(* Logix 5000 AddOnInstructionDefinition export Banner_TL50_Param_v4; software revision 32.00 *)

TYPE Banner_IOL_Port_v4 :   // UDT that has all of the data items necessary to communicate with a specific Port on a IO-Link Master
STRUCT
   Port_Controlled : INT;   // Each bit represents a port on an IO-Link Master. Set to 1 to tell AOI to control that port.
   Port_Activate : INT;   // Each bit represents a port on an IO-Link Master. When ON that port will process any commands in queue.
   Port_Read : INT;   // Each bit represents a port on an IO-Link Master. Used to determine when device AOI has requested a Read command.
   Port_Write : INT;   // Each bit represents a port on an IO-Link Master. Used to determine when device AOI has requested a Write command.
   Port_RW_Complete : INT;   // Each bit represents a port on an IO-Link Master. Tells device AOI that Read or Write request has been completed.
   Port_Device_Read : INT;
   Data_Transfer : SINT[190];   // Array to transfer data from IO-Master to device AOIs.
END_STRUCT
END_TYPE

TYPE Banner_TL50_RD_v2 :   // All of the read parameters for a TL50.
STRUCT
   Master_Cycle_Time : INT;
   Min_Cycle_Time : INT;
   M_Sequence_Capability : INT;
   IO_Link_Version_ID : INT;
   Process_Data_Input_Length : INT;
   Process_Data_Output_Length : INT;
   Combined_Vendor_ID : DINT;   // IO-Link Vendor ID
   Vendor_ID1 : INT;
   Vendor_ID2 : INT;
   Combined_Device_ID : DINT;   // IO-Link Device ID
   Device_ID1 : INT;
   Device_ID2 : INT;
   Device_ID3 : INT;
   Serial_Number : STRING;
   Segment_1_State : SINT;   // State of the TL50 Segment. 0 = Off, 1 = On, 2 = Flashing
   Segment_2_State : SINT;   // State of the TL50 Segment. 0 = Off, 1 = On, 2 = Flashing
   Segment_3_State : SINT;   // State of the TL50 Segment. 0 = Off, 1 = On, 2 = Flashing
   Segment_4_State : SINT;   // State of the TL50 Segment. 0 = Off, 1 = On, 2 = Flashing
   Segment_5_State : SINT;   // State of the TL50 Segment. 0 = Off, 1 = On, 2 = Flashing
   Segment_6_State : SINT;   // State of the TL50 Segment. 0 = Off, 1 = On, 2 = Flashing
   Segment_7_State : SINT;   // State of the TL50 Segment. 0 = Off, 1 = On, 2 = Flashing
   Number_of_Segments : INT;   // Number of Segment detected for the TL50.
END_STRUCT
END_TYPE

TYPE Banner_TL50_v2 :   // All of the parameters for a TL50.
STRUCT
   Initial_Global_Read : BOOL;   // Determines if all of the IO-Link data has been read into the PLC yet
   Command : INT;   // Value placed in here will activate a read or write to a specifc IO-Link Index
   Read_Data : Banner_TL50_RD_v2;   // Read Only Data
   Write_Data : Banner_TL50_WD_v2;   // Write Data
   Archive : Banner_TL50_WD_v2;   // Archive Data
   Reset : BOOL;   // Resets AOI. This will force a complete parameter read of the sensor.
END_STRUCT
END_TYPE

TYPE Banner_TL50_WD_v2 :   // UDT that stores the Write Data for a TL50.
STRUCT
   System_Command : INT;   // See IODD file for list of commands that can be activated via the System Command interface
   Parameter_Access_Lock : SINT;   // Write access to all parameters is prohibited while value is 1. Only this parameter can be adjusted when value is 1.
   Data_Storage_Lock : SINT;   // Automatic data storage is disabled when this value is equal to 1. Read access is not affected.
   Local_Parameterization_Lock : SINT;   // Parameterization via local control elements on device is disabled.
   Local_User_Interface_Lock : SINT;   // Operation of local user interface is disabled.
   Flashing_Frequency_1 : DINT;   // Value in .1 Hz increments.
   Flashing_Frequency_2 : DINT;   // Value in .1 Hz increments.
   Flashing_Frequency_3 : DINT;   // Value in .1 Hz increments.
   Flashing_Frequency_4 : DINT;   // Value in .1 Hz increments.
   Flashing_Frequency_5 : DINT;   // Value in .1 Hz increments.
   Flashing_Frequency_6 : DINT;   // Value in .1 Hz increments.
   Flashing_Frequency_7 : DINT;   // Value in .1 Hz increments.
END_STRUCT
END_TYPE

ADD_ON_INSTRUCTION Banner_TL50_Param_v4   (* revision 4.0, vendor Banner Engineering *)
// AOI to read and write parameter data to an IO-Link TL50.
VAR_IN_OUT
   TL50 : Banner_TL50_v2; {required}
   Port_Data : Banner_IOL_Port_v4; {required}
END_VAR
VAR_INPUT
   Port : DINT; {required}
END_VAR
VAR
   Local_Control : DINT; {access None}
   Global_Read_Command_Value : INT; {access None}
   Global_Write_Command_Value : INT; {access None}
   Error_Generated : BOOL; {access None}
   Command_Being_Processed : BOOL; {access None}
   Index_Write_Inprocess : INT; {access None}
   Index_Write_Control : INT; {access None}
   Update_Archive : BOOL; {access None}
   Inprocess_Index : DINT; {access None}
END_VAR

ROUTINE Logic   (* ladder *)
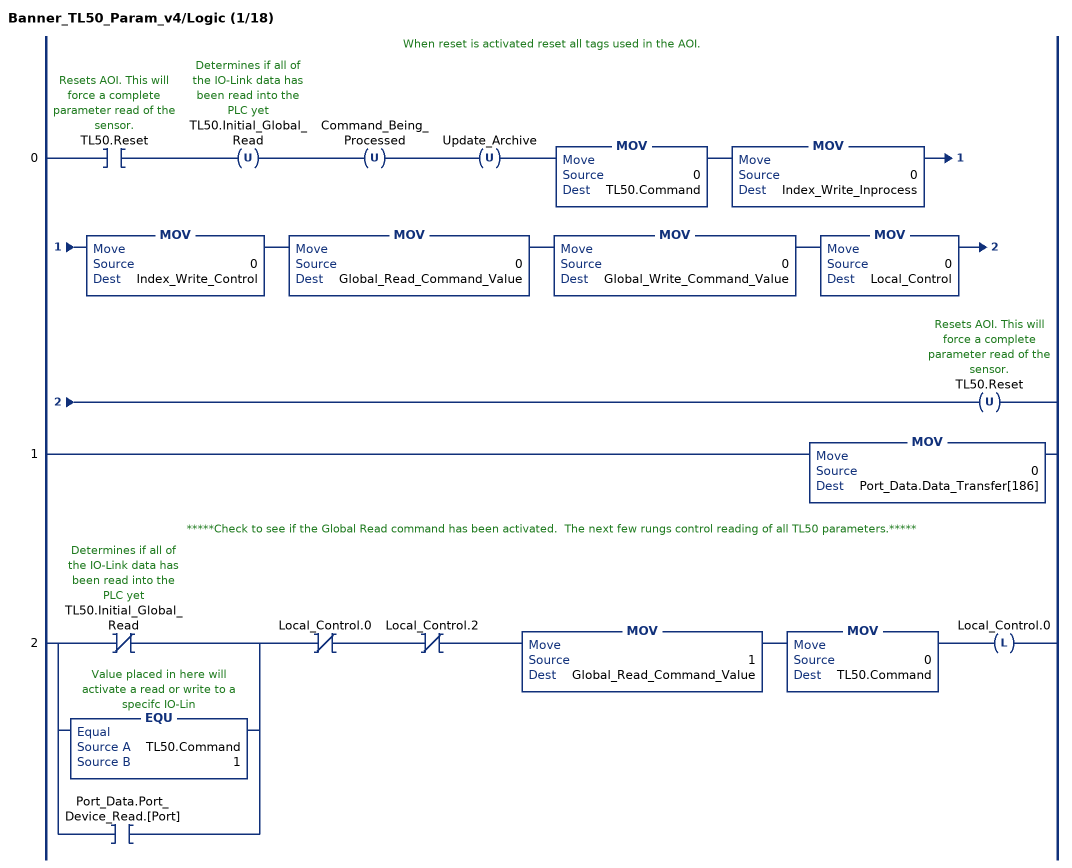
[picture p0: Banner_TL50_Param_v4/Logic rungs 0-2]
   // When reset is activated reset all tags used in the AOI.
   0: XIC(TL50.Reset)OTU(TL50.Initial_Global_Read)OTU(Command_Being_Processed)OTU(Update_Archive)MOV(0,TL50.Command)MOV(0,Index_Write_Inprocess)MOV(0,Index_Write_Control)MOV(0,Global_Read_Command_Value)MOV(0,Global_Write_Command_Value)MOV(0,Local_Control)OTU(TL50.Reset);
   1: MOV(0,Port_Data.Data_Transfer[186]);
   // *****Check to see if the Global Read command has been activated.  The next few rungs control reading of all TL50 parameters.*****
   2: [XIO(TL50.Initial_Global_Read) ,EQU(TL50.Command,1) ,XIC(Port_Data.Port_Device_Read.[Port]) ]XIO(Local_Control.0)XIO(Local_Control.2)MOV(1,Global_Read_Command_Value)MOV(0,TL50.Command)OTL(Local_Control.0);
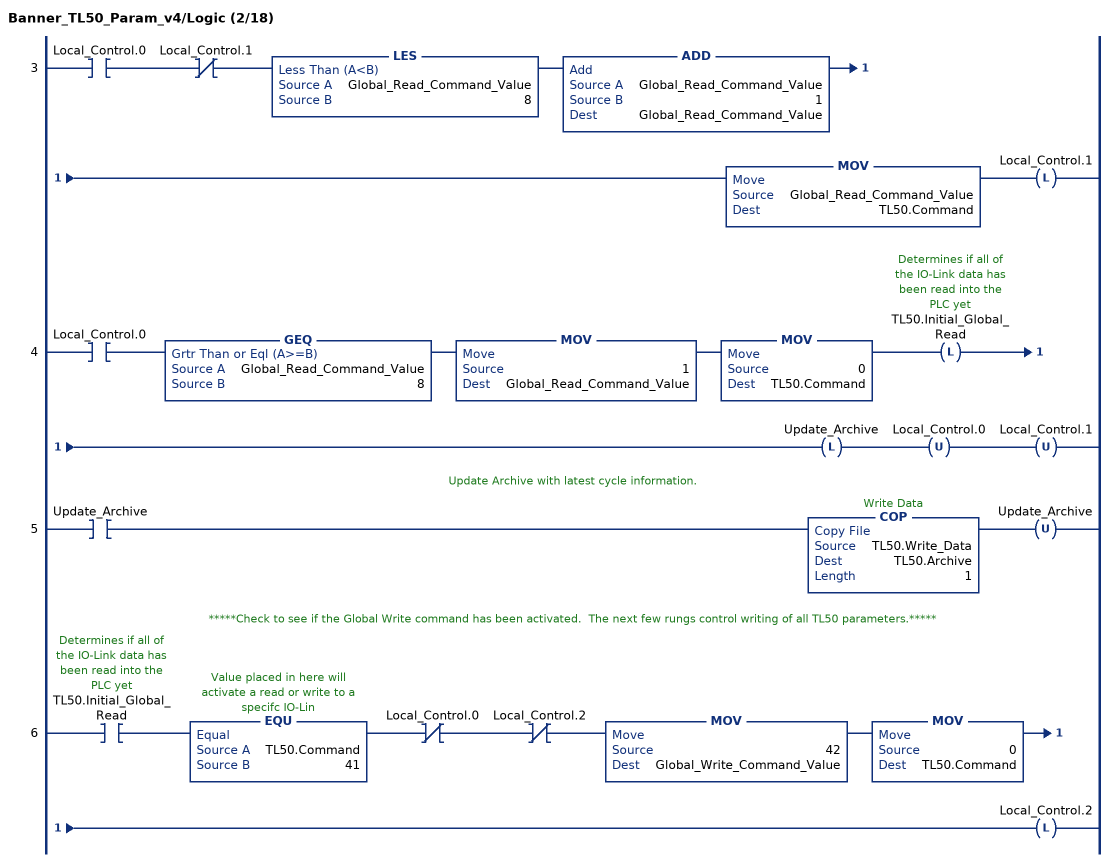
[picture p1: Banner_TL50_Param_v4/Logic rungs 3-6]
   3: XIC(Local_Control.0)XIO(Local_Control.1)LES(Global_Read_Command_Value,8)ADD(Global_Read_Command_Value,1,Global_Read_Command_Value)MOV(Global_Read_Command_Value,TL50.Command)OTL(Local_Control.1);
   4: XIC(Local_Control.0)GEQ(Global_Read_Command_Value,8)MOV(1,Global_Read_Command_Value)MOV(0,TL50.Command)OTL(TL50.Initial_Global_Read)OTL(Update_Archive)OTU(Local_Control.0)OTU(Local_Control.1);
   // Update Archive with latest cycle information.
   5: XIC(Update_Archive)COP(TL50.Write_Data,TL50.Archive,1)OTU(Update_Archive);
   // *****Check to see if the Global Write command has been activated.  The next few rungs control writing of all TL50 parameters.*****
   6: XIC(TL50.Initial_Global_Read)EQU(TL50.Command,41)XIO(Local_Control.0)XIO(Local_Control.2)MOV(42,Global_Write_Command_Value)MOV(0,TL50.Command)OTL(Local_Control.2);
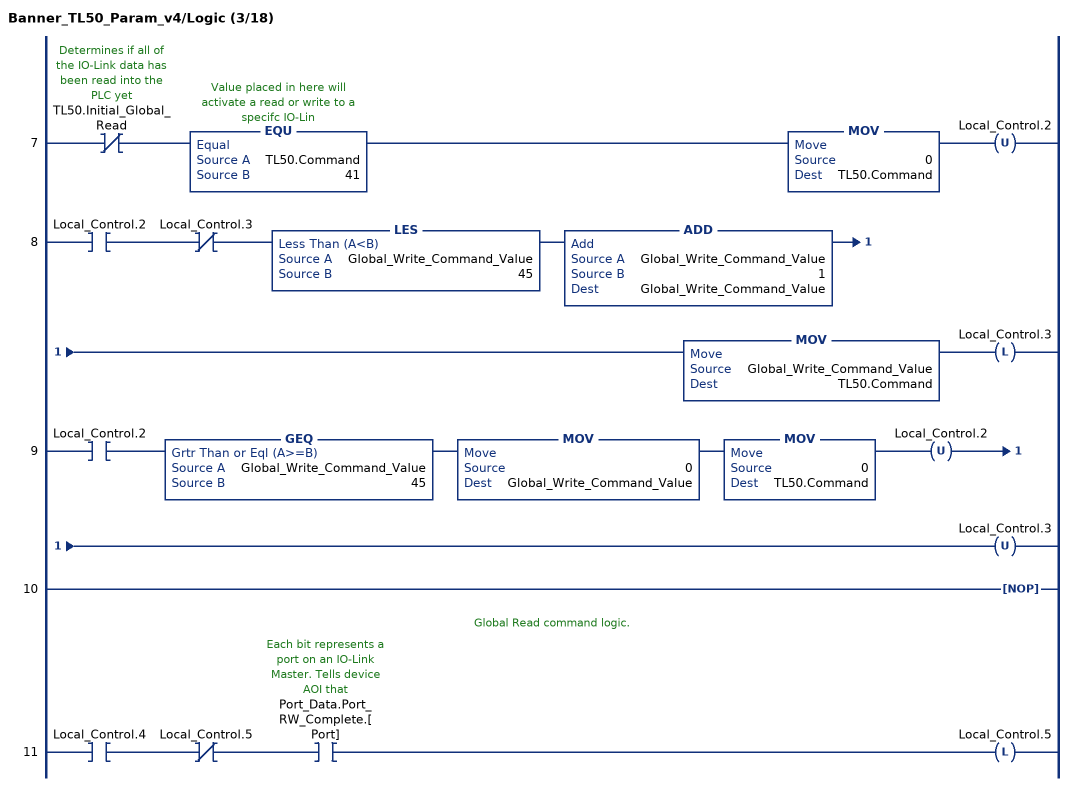
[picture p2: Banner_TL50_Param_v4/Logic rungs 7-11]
   7: XIO(TL50.Initial_Global_Read)EQU(TL50.Command,41)MOV(0,TL50.Command)OTU(Local_Control.2);
   8: XIC(Local_Control.2)XIO(Local_Control.3)LES(Global_Write_Command_Value,45)ADD(Global_Write_Command_Value,1,Global_Write_Command_Value)MOV(Global_Write_Command_Value,TL50.Command)OTL(Local_Control.3);
   9: XIC(Local_Control.2)GEQ(Global_Write_Command_Value,45)MOV(0,Global_Write_Command_Value)MOV(0,TL50.Command)OTU(Local_Control.2)OTU(Local_Control.3);
   10: NOP();
   // Global Read command logic.
   11: XIC(Local_Control.4)XIO(Local_Control.5)XIC(Port_Data.Port_RW_Complete.[Port])OTL(Local_Control.5);
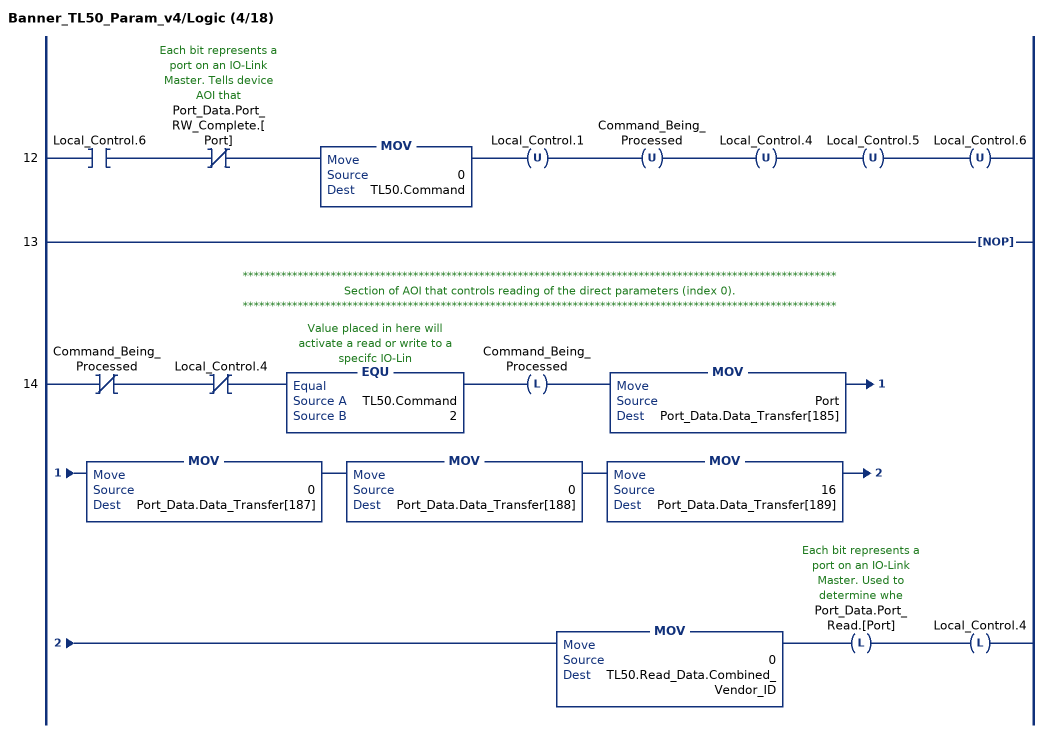
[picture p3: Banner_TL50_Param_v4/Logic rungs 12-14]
   12: XIC(Local_Control.6)XIO(Port_Data.Port_RW_Complete.[Port])MOV(0,TL50.Command)OTU(Local_Control.1)OTU(Command_Being_Processed)OTU(Local_Control.4)OTU(Local_Control.5)OTU(Local_Control.6);
   13: NOP();
   // ************************************************************************************************************
   // Section of AOI that controls reading of the direct parameters (index 0).
   // ************************************************************************************************************
   14: XIO(Command_Being_Processed)XIO(Local_Control.4)EQU(TL50.Command,2)OTL(Command_Being_Processed)MOV(Port,Port_Data.Data_Transfer[185])MOV(0,Port_Data.Data_Transfer[187])MOV(0,Port_Data.Data_Transfer[188])MOV(16,Port_Data.Data_Transfer[189])MOV(0,TL50.Read_Data.Combined_Vendor_ID)OTL(Port_Data.Port_Read.[Port])OTL(Local_Control.4);
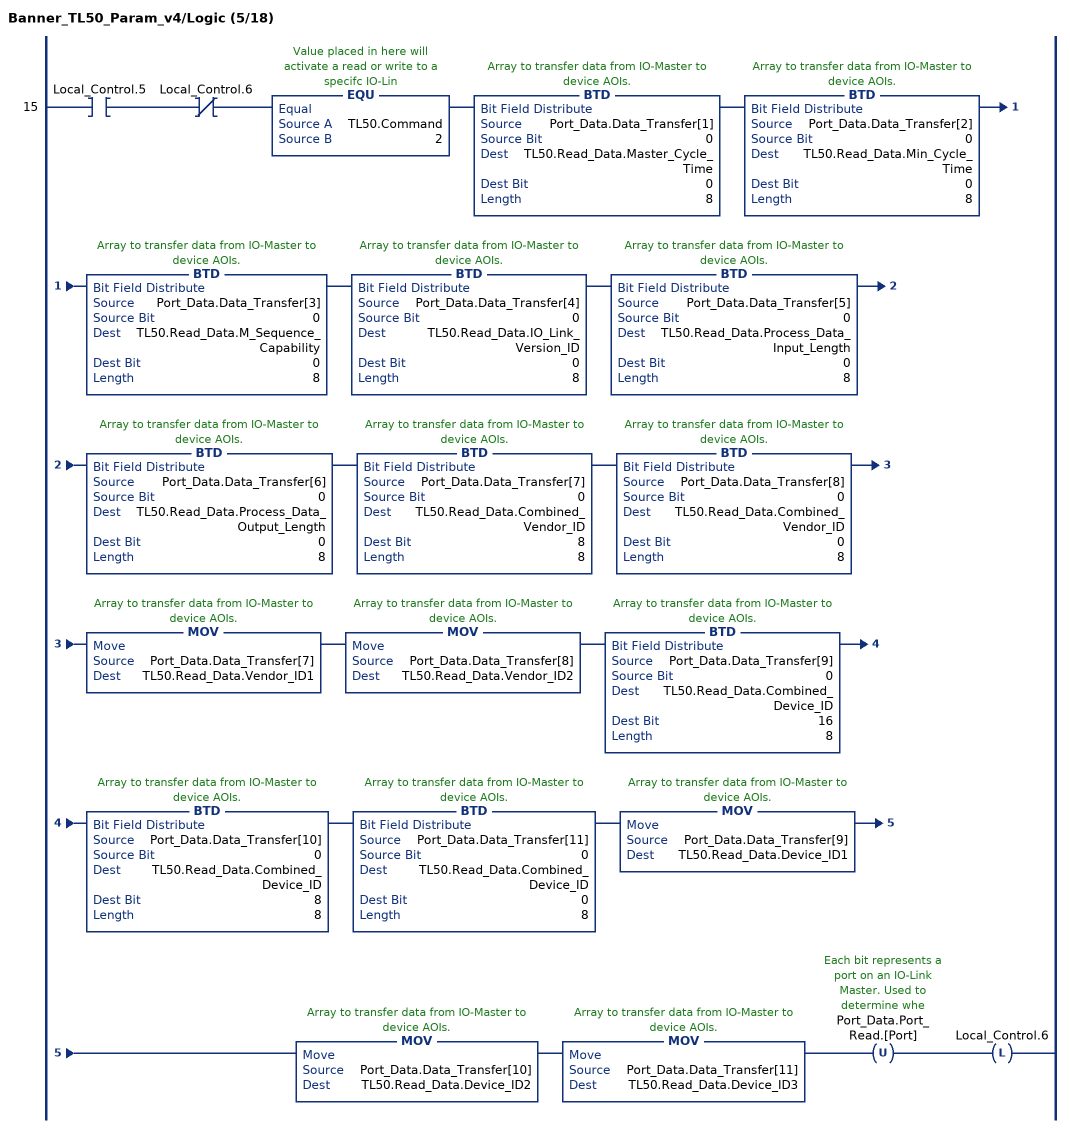
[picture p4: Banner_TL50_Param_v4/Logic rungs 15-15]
   15: XIC(Local_Control.5)XIO(Local_Control.6)EQU(TL50.Command,2)BTD(Port_Data.Data_Transfer[1],0,TL50.Read_Data.Master_Cycle_Time,0,8)BTD(Port_Data.Data_Transfer[2],0,TL50.Read_Data.Min_Cycle_Time,0,8)BTD(Port_Data.Data_Transfer[3],0,TL50.Read_Data.M_Sequence_Capability,0,8)BTD(Port_Data.Data_Transfer[4],0,TL50.Read_Data.IO_Link_Version_ID,0,8)BTD(Port_Data.Data_Transfer[5],0,TL50.Read_Data.Process_Data_Input_Length,0,8)BTD(Port_Data.Data_Transfer[6],0,TL50.Read_Data.Process_Data_Output_Length,0,8)BTD(Port_Data.Data_Transfer[7],0,TL50.Read_Data.Combined_Vendor_ID,8,8)BTD(Port_Data.Data_Transfer[8],0,TL50.Read_Data.Combined_Vendor_ID,0,8)MOV(Port_Data.Data_Transfer[7],TL50.Read_Data.Vendor_ID1)MOV(Port_Data.Data_Transfer[8],TL50.Read_Data.Vendor_ID2)BTD(Port_Data.Data_Transfer[9],0,TL50.Read_Data.Combined_Device_ID,16,8)BTD(Port_Data.Data_Transfer[10],0,TL50.Read_Data.Combined_Device_ID,8,8)BTD(Port_Data.Data_Transfer[11],0,TL50.Read_Data.Combined_Device_ID,0,8)MOV(Port_Data.Data_Transfer[9],TL50.Read_Data.Device_ID1)MOV(Port_Data.Data_Transfer[10],TL50.Read_Data.Device_ID2)MOV(Port_Data.Data_Transfer[11],TL50.Read_Data.Device_ID3)OTU(Port_Data.Port_Read.[Port])OTL(Local_Control.6);
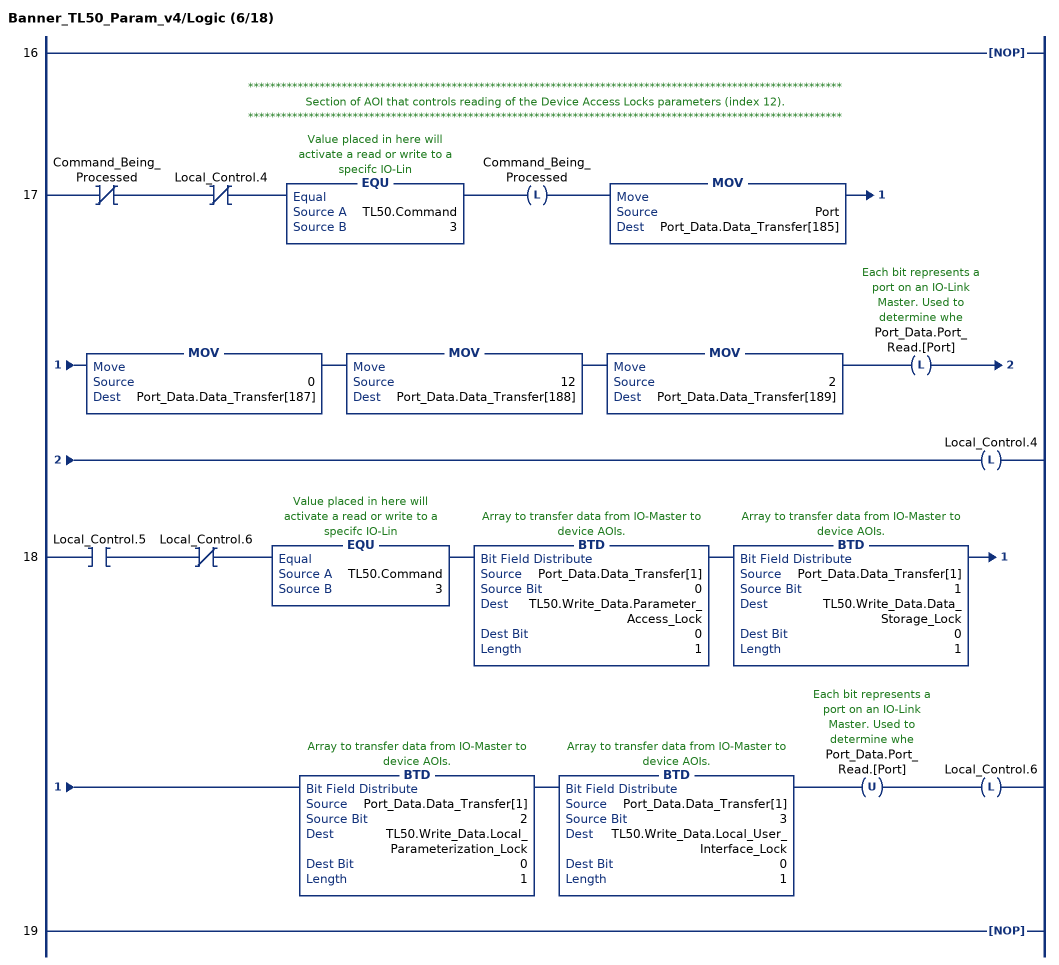
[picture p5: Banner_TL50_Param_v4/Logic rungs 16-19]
   16: NOP();
   // ************************************************************************************************************
   // Section of AOI that controls reading of the Device Access Locks parameters (index 12).
   // ************************************************************************************************************
   17: XIO(Command_Being_Processed)XIO(Local_Control.4)EQU(TL50.Command,3)OTL(Command_Being_Processed)MOV(Port,Port_Data.Data_Transfer[185])MOV(0,Port_Data.Data_Transfer[187])MOV(12,Port_Data.Data_Transfer[188])MOV(2,Port_Data.Data_Transfer[189])OTL(Port_Data.Port_Read.[Port])OTL(Local_Control.4);
   18: XIC(Local_Control.5)XIO(Local_Control.6)EQU(TL50.Command,3)BTD(Port_Data.Data_Transfer[1],0,TL50.Write_Data.Parameter_Access_Lock,0,1)BTD(Port_Data.Data_Transfer[1],1,TL50.Write_Data.Data_Storage_Lock,0,1)BTD(Port_Data.Data_Transfer[1],2,TL50.Write_Data.Local_Parameterization_Lock,0,1)BTD(Port_Data.Data_Transfer[1],3,TL50.Write_Data.Local_User_Interface_Lock,0,1)OTU(Port_Data.Port_Read.[Port])OTL(Local_Control.6);
   19: NOP();
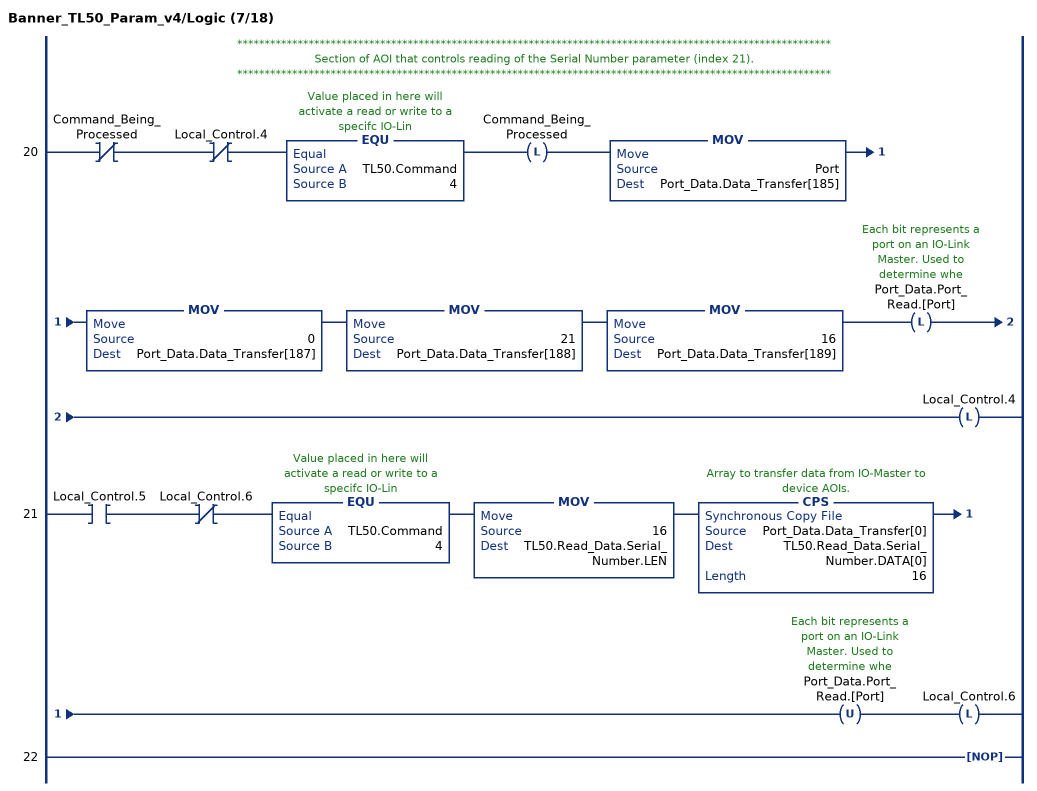
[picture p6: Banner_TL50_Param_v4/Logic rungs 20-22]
   // ************************************************************************************************************
   // Section of AOI that controls reading of the Serial Number parameter (index 21).
   // ************************************************************************************************************
   20: XIO(Command_Being_Processed)XIO(Local_Control.4)EQU(TL50.Command,4)OTL(Command_Being_Processed)MOV(Port,Port_Data.Data_Transfer[185])MOV(0,Port_Data.Data_Transfer[187])MOV(21,Port_Data.Data_Transfer[188])MOV(16,Port_Data.Data_Transfer[189])OTL(Port_Data.Port_Read.[Port])OTL(Local_Control.4);
   21: XIC(Local_Control.5)XIO(Local_Control.6)EQU(TL50.Command,4)MOV(16,TL50.Read_Data.Serial_Number.LEN)CPS(Port_Data.Data_Transfer[0],TL50.Read_Data.Serial_Number.DATA[0],16)OTU(Port_Data.Port_Read.[Port])OTL(Local_Control.6);
   22: NOP();
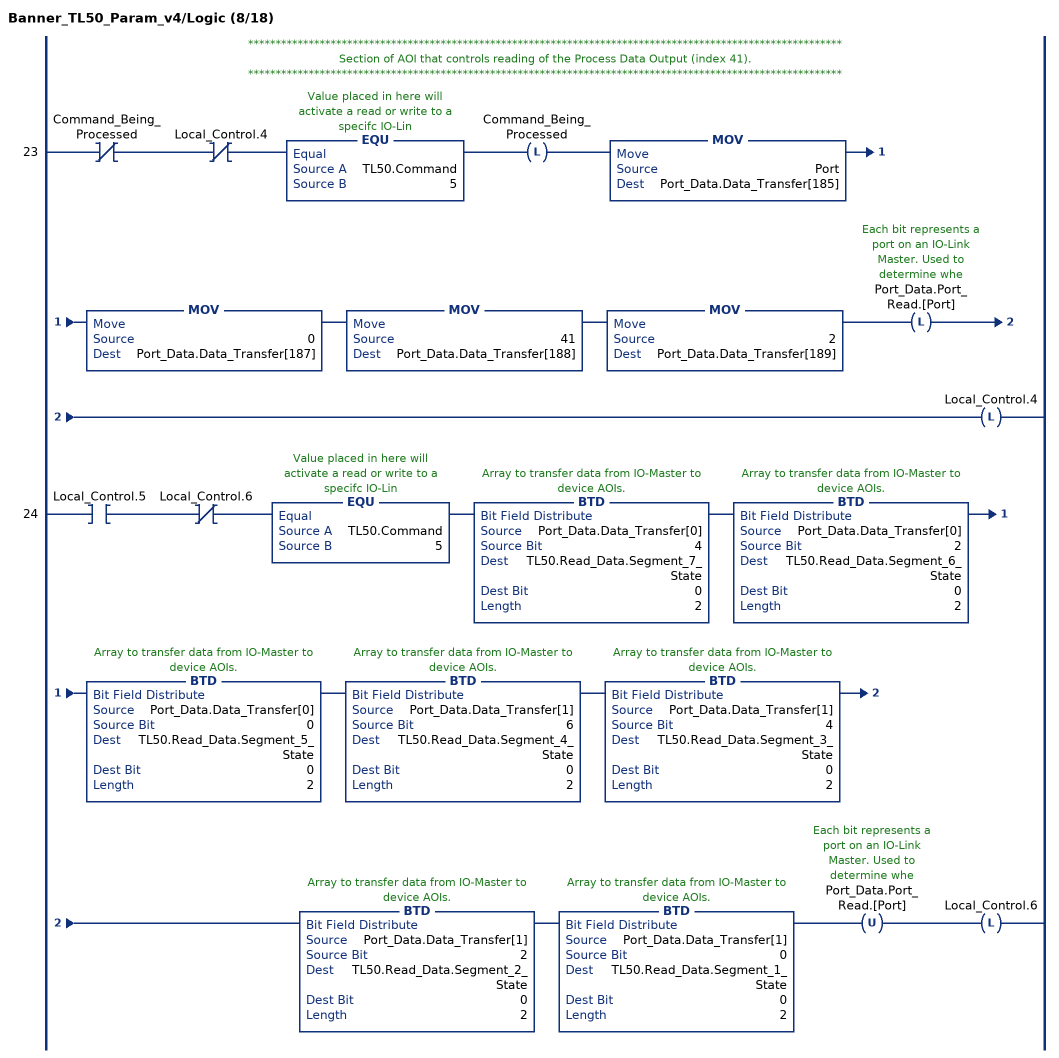
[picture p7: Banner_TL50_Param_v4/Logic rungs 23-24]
   // ************************************************************************************************************
   // Section of AOI that controls reading of the Process Data Output (index 41).
   // ************************************************************************************************************
   23: XIO(Command_Being_Processed)XIO(Local_Control.4)EQU(TL50.Command,5)OTL(Command_Being_Processed)MOV(Port,Port_Data.Data_Transfer[185])MOV(0,Port_Data.Data_Transfer[187])MOV(41,Port_Data.Data_Transfer[188])MOV(2,Port_Data.Data_Transfer[189])OTL(Port_Data.Port_Read.[Port])OTL(Local_Control.4);
   24: XIC(Local_Control.5)XIO(Local_Control.6)EQU(TL50.Command,5)BTD(Port_Data.Data_Transfer[0],4,TL50.Read_Data.Segment_7_State,0,2)BTD(Port_Data.Data_Transfer[0],2,TL50.Read_Data.Segment_6_State,0,2)BTD(Port_Data.Data_Transfer[0],0,TL50.Read_Data.Segment_5_State,0,2)BTD(Port_Data.Data_Transfer[1],6,TL50.Read_Data.Segment_4_State,0,2)BTD(Port_Data.Data_Transfer[1],4,TL50.Read_Data.Segment_3_State,0,2)BTD(Port_Data.Data_Transfer[1],2,TL50.Read_Data.Segment_2_State,0,2)BTD(Port_Data.Data_Transfer[1],0,TL50.Read_Data.Segment_1_State,0,2)OTU(Port_Data.Port_Read.[Port])OTL(Local_Control.6);
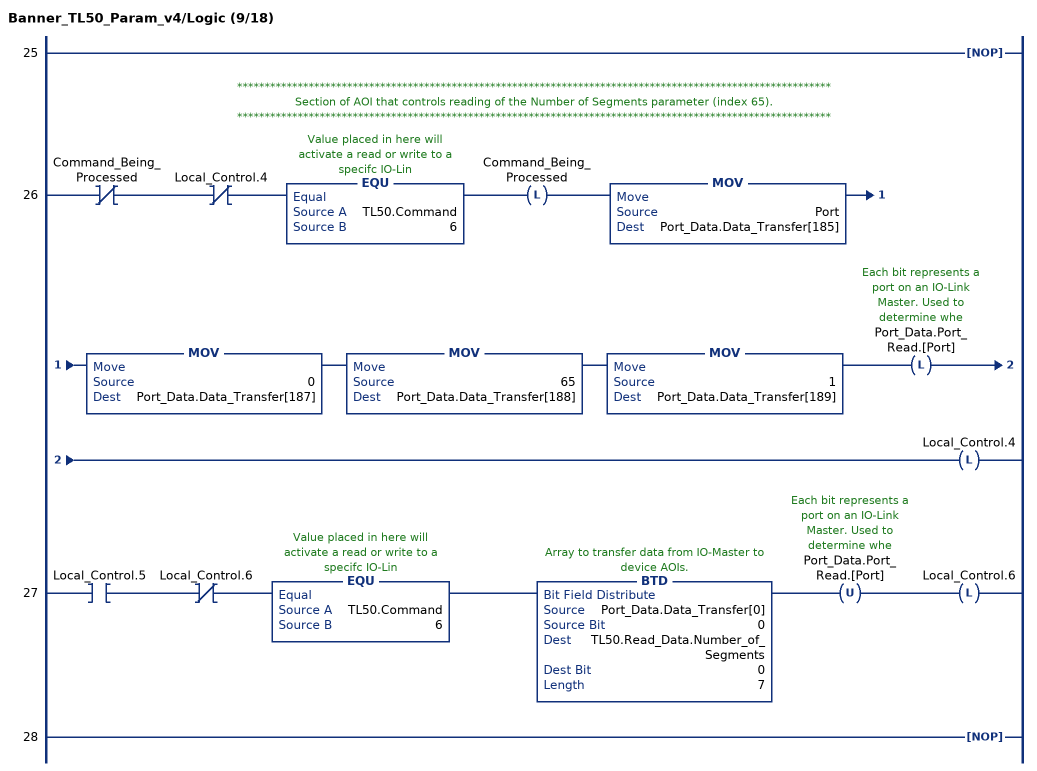
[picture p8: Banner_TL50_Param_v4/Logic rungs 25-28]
   25: NOP();
   // ************************************************************************************************************
   // Section of AOI that controls reading of the Number of Segments parameter (index 65).
   // ************************************************************************************************************
   26: XIO(Command_Being_Processed)XIO(Local_Control.4)EQU(TL50.Command,6)OTL(Command_Being_Processed)MOV(Port,Port_Data.Data_Transfer[185])MOV(0,Port_Data.Data_Transfer[187])MOV(65,Port_Data.Data_Transfer[188])MOV(1,Port_Data.Data_Transfer[189])OTL(Port_Data.Port_Read.[Port])OTL(Local_Control.4);
   27: XIC(Local_Control.5)XIO(Local_Control.6)EQU(TL50.Command,6)BTD(Port_Data.Data_Transfer[0],0,TL50.Read_Data.Number_of_Segments,0,7)OTU(Port_Data.Port_Read.[Port])OTL(Local_Control.6);
   28: NOP();
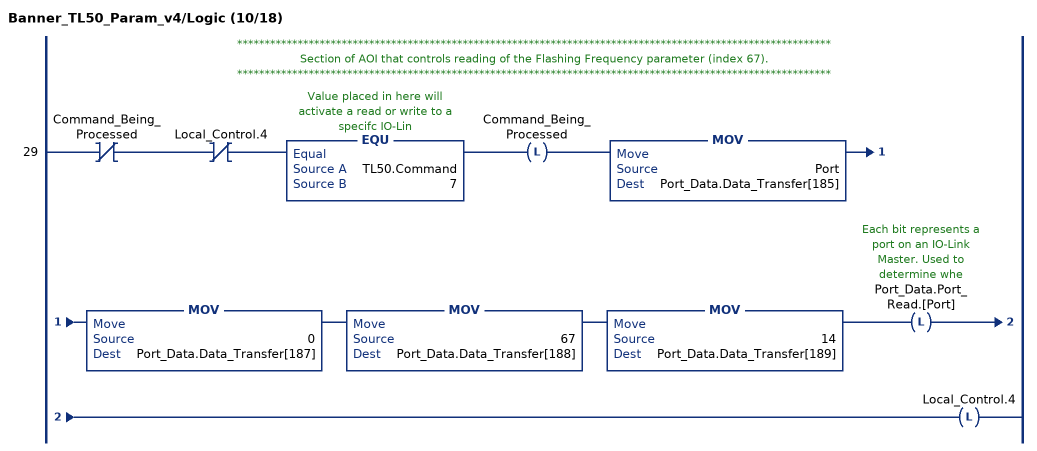
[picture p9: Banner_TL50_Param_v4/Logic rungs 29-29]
   // ************************************************************************************************************
   // Section of AOI that controls reading of the Flashing Frequency parameter (index 67).
   // ************************************************************************************************************
   29: XIO(Command_Being_Processed)XIO(Local_Control.4)EQU(TL50.Command,7)OTL(Command_Being_Processed)MOV(Port,Port_Data.Data_Transfer[185])MOV(0,Port_Data.Data_Transfer[187])MOV(67,Port_Data.Data_Transfer[188])MOV(14,Port_Data.Data_Transfer[189])OTL(Port_Data.Port_Read.[Port])OTL(Local_Control.4);
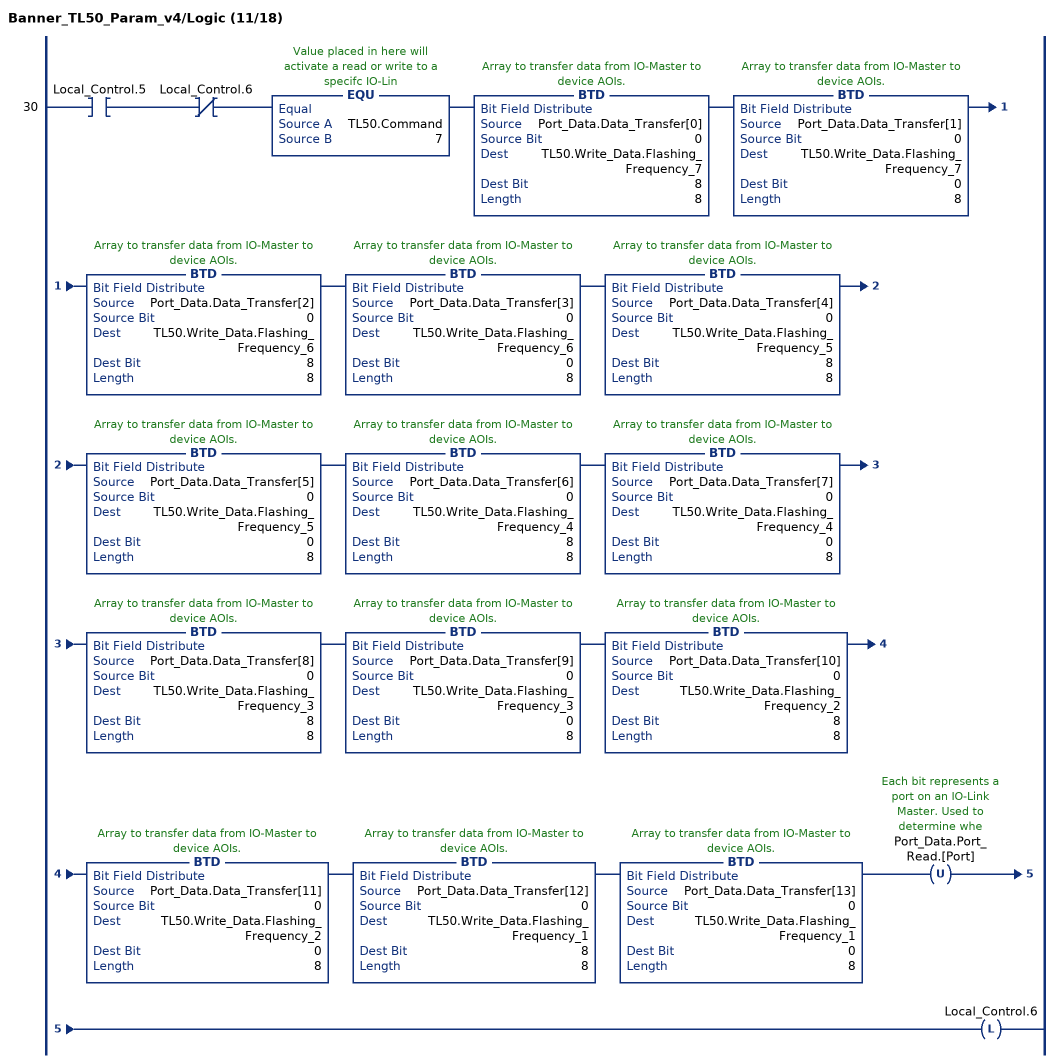
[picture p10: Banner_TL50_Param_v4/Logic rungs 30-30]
   30: XIC(Local_Control.5)XIO(Local_Control.6)EQU(TL50.Command,7)BTD(Port_Data.Data_Transfer[0],0,TL50.Write_Data.Flashing_Frequency_7,8,8)BTD(Port_Data.Data_Transfer[1],0,TL50.Write_Data.Flashing_Frequency_7,0,8)BTD(Port_Data.Data_Transfer[2],0,TL50.Write_Data.Flashing_Frequency_6,8,8)BTD(Port_Data.Data_Transfer[3],0,TL50.Write_Data.Flashing_Frequency_6,0,8)BTD(Port_Data.Data_Transfer[4],0,TL50.Write_Data.Flashing_Frequency_5,8,8)BTD(Port_Data.Data_Transfer[5],0,TL50.Write_Data.Flashing_Frequency_5,0,8)BTD(Port_Data.Data_Transfer[6],0,TL50.Write_Data.Flashing_Frequency_4,8,8)BTD(Port_Data.Data_Transfer[7],0,TL50.Write_Data.Flashing_Frequency_4,0,8)BTD(Port_Data.Data_Transfer[8],0,TL50.Write_Data.Flashing_Frequency_3,8,8)BTD(Port_Data.Data_Transfer[9],0,TL50.Write_Data.Flashing_Frequency_3,0,8)BTD(Port_Data.Data_Transfer[10],0,TL50.Write_Data.Flashing_Frequency_2,8,8)BTD(Port_Data.Data_Transfer[11],0,TL50.Write_Data.Flashing_Frequency_2,0,8)BTD(Port_Data.Data_Transfer[12],0,TL50.Write_Data.Flashing_Frequency_1,8,8)BTD(Port_Data.Data_Transfer[13],0,TL50.Write_Data.Flashing_Frequency_1,0,8)OTU(Port_Data.Port_Read.[Port])OTL(Local_Control.6);
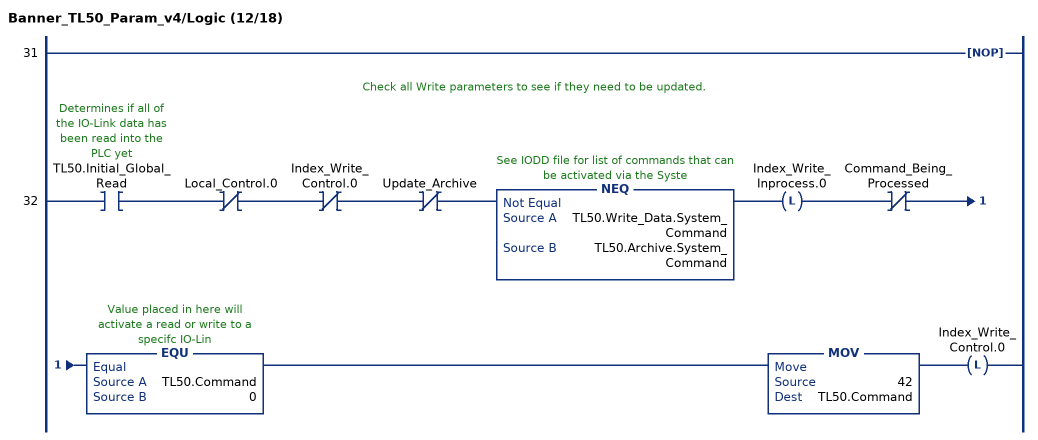
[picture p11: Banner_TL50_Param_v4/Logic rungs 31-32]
   31: NOP();
   // Check all Write parameters to see if they need to be updated.
   32: XIC(TL50.Initial_Global_Read)XIO(Local_Control.0)XIO(Index_Write_Control.0)XIO(Update_Archive)NEQ(TL50.Write_Data.System_Command,TL50.Archive.System_Command)OTL(Index_Write_Inprocess.0)XIO(Command_Being_Processed)EQU(TL50.Command,0)MOV(42,TL50.Command)OTL(Index_Write_Control.0);
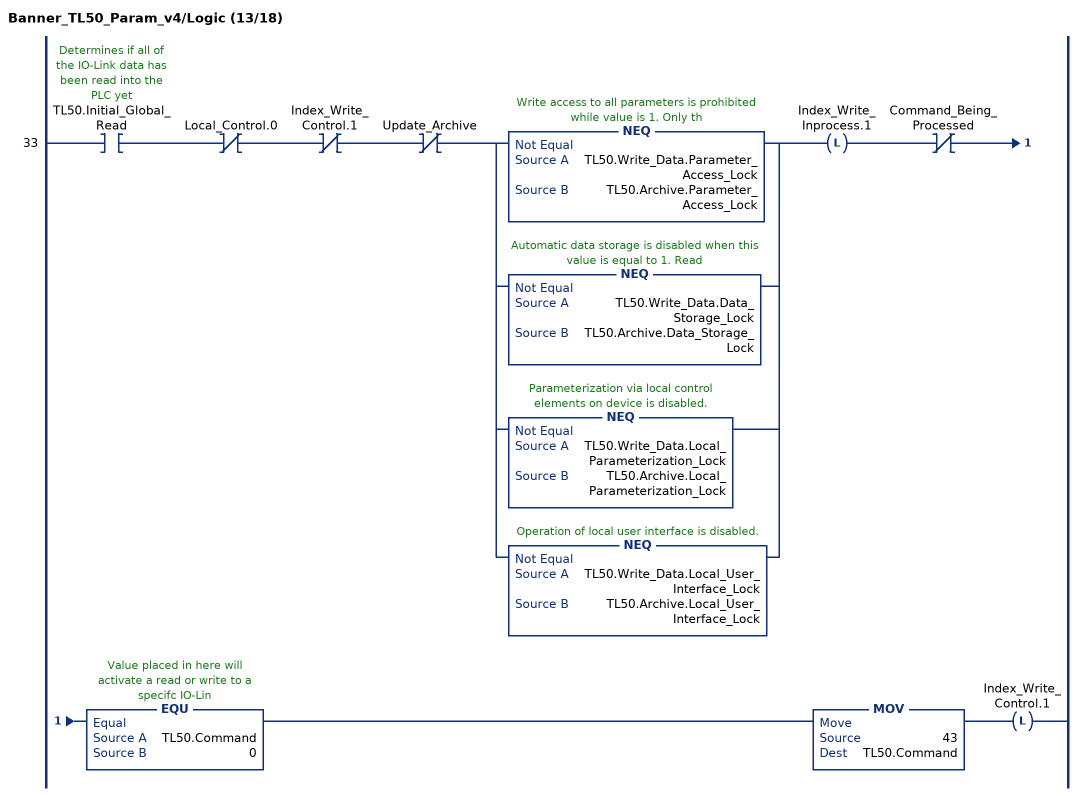
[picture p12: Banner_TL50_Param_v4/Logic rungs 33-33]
   33: XIC(TL50.Initial_Global_Read)XIO(Local_Control.0)XIO(Index_Write_Control.1)XIO(Update_Archive)[NEQ(TL50.Write_Data.Parameter_Access_Lock,TL50.Archive.Parameter_Access_Lock) ,NEQ(TL50.Write_Data.Data_Storage_Lock,TL50.Archive.Data_Storage_Lock) ,NEQ(TL50.Write_Data.Local_Parameterization_Lock,TL50.Archive.Local_Parameterization_Lock) ,NEQ(TL50.Write_Data.Local_User_Interface_Lock,TL50.Archive.Local_User_Interface_Lock) ]OTL(Index_Write_Inprocess.1)XIO(Command_Being_Processed)EQU(TL50.Command,0)MOV(43,TL50.Command)OTL(Index_Write_Control.1);
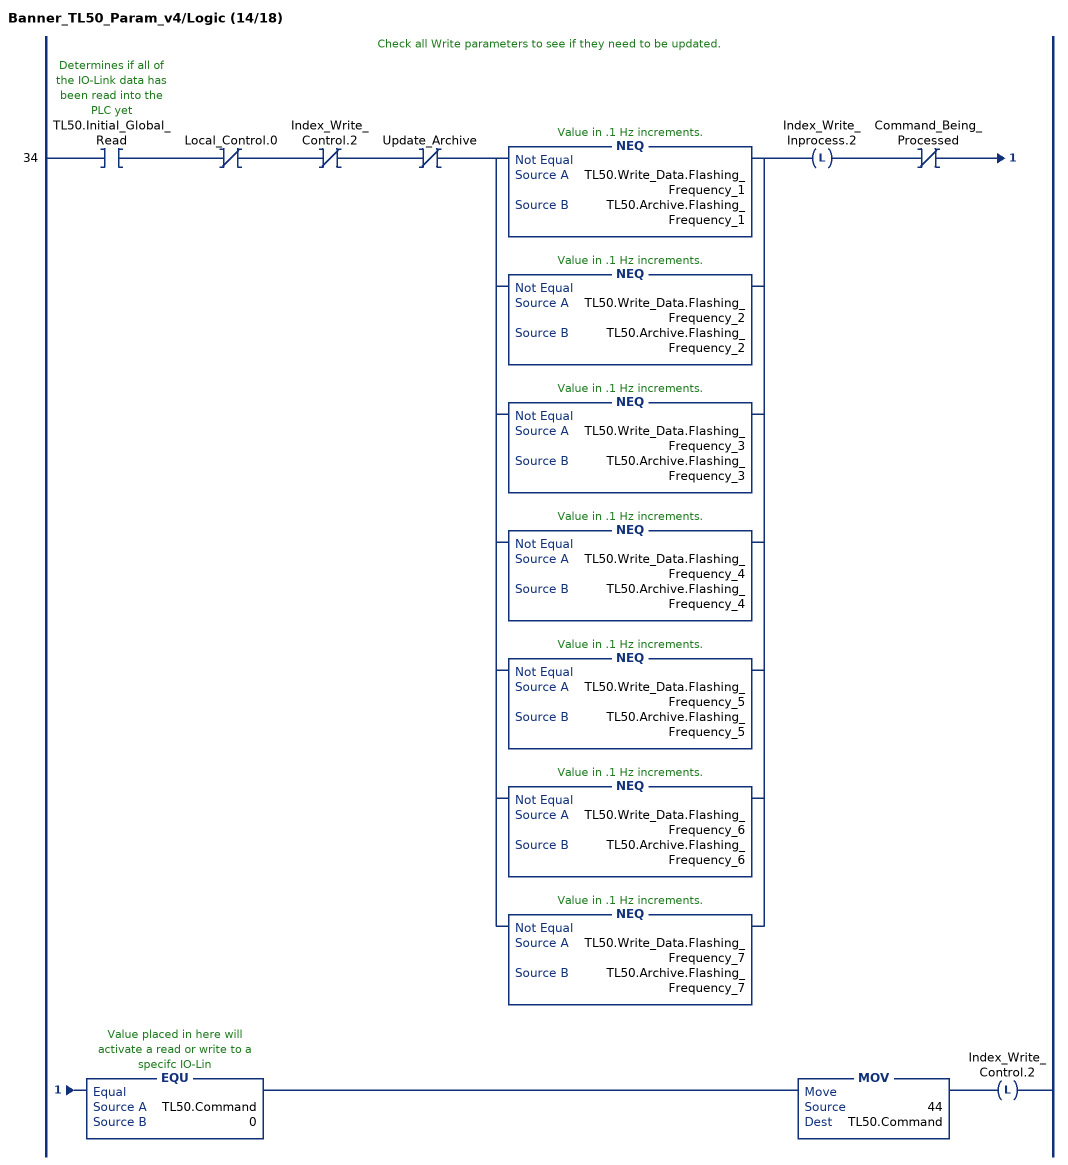
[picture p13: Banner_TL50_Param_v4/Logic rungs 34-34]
   // Check all Write parameters to see if they need to be updated.
   34: XIC(TL50.Initial_Global_Read)XIO(Local_Control.0)XIO(Index_Write_Control.2)XIO(Update_Archive)[NEQ(TL50.Write_Data.Flashing_Frequency_1,TL50.Archive.Flashing_Frequency_1) ,NEQ(TL50.Write_Data.Flashing_Frequency_2,TL50.Archive.Flashing_Frequency_2) ,NEQ(TL50.Write_Data.Flashing_Frequency_3,TL50.Archive.Flashing_Frequency_3) ,NEQ(TL50.Write_Data.Flashing_Frequency_4,TL50.Archive.Flashing_Frequency_4) ,NEQ(TL50.Write_Data.Flashing_Frequency_5,TL50.Archive.Flashing_Frequency_5) ,NEQ(TL50.Write_Data.Flashing_Frequency_6,TL50.Archive.Flashing_Frequency_6) ,NEQ(TL50.Write_Data.Flashing_Frequency_7,TL50.Archive.Flashing_Frequency_7) ]OTL(Index_Write_Inprocess.2)XIO(Command_Being_Processed)EQU(TL50.Command,0)MOV(44,TL50.Command)OTL(Index_Write_Control.2);
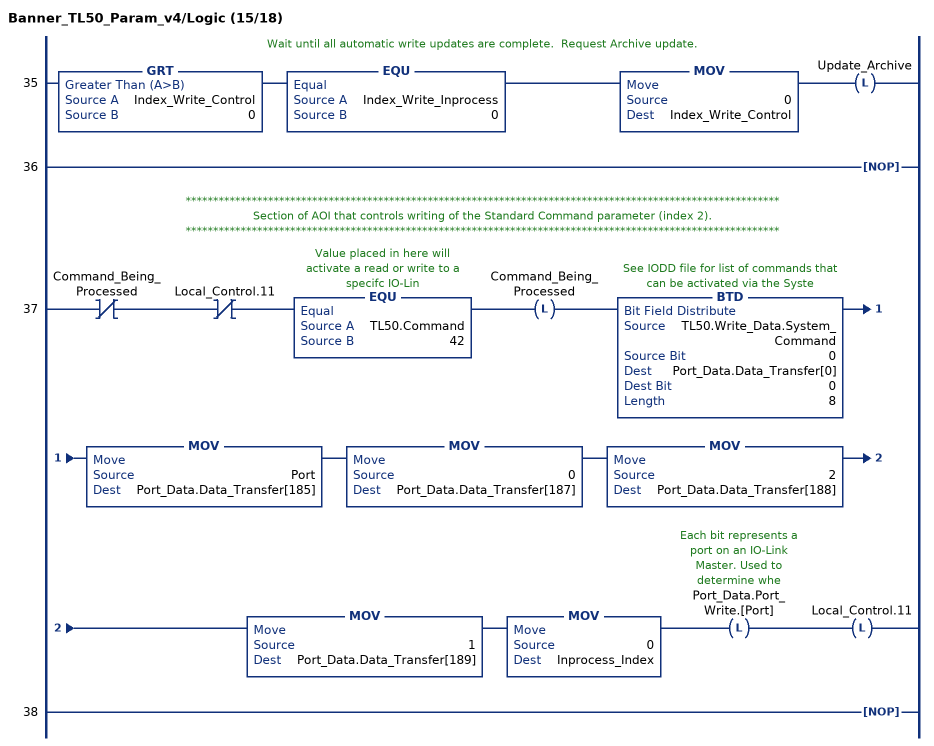
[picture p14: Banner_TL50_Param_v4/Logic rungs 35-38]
   // Wait until all automatic write updates are complete.  Request Archive update.
   35: GRT(Index_Write_Control,0)EQU(Index_Write_Inprocess,0)MOV(0,Index_Write_Control)OTL(Update_Archive);
   36: NOP();
   // ************************************************************************************************************
   // Section of AOI that controls writing of the Standard Command parameter (index 2).
   // ************************************************************************************************************
   37: XIO(Command_Being_Processed)XIO(Local_Control.11)EQU(TL50.Command,42)OTL(Command_Being_Processed)BTD(TL50.Write_Data.System_Command,0,Port_Data.Data_Transfer[0],0,8)MOV(Port,Port_Data.Data_Transfer[185])MOV(0,Port_Data.Data_Transfer[187])MOV(2,Port_Data.Data_Transfer[188])MOV(1,Port_Data.Data_Transfer[189])MOV(0,Inprocess_Index)OTL(Port_Data.Port_Write.[Port])OTL(Local_Control.11);
   38: NOP();
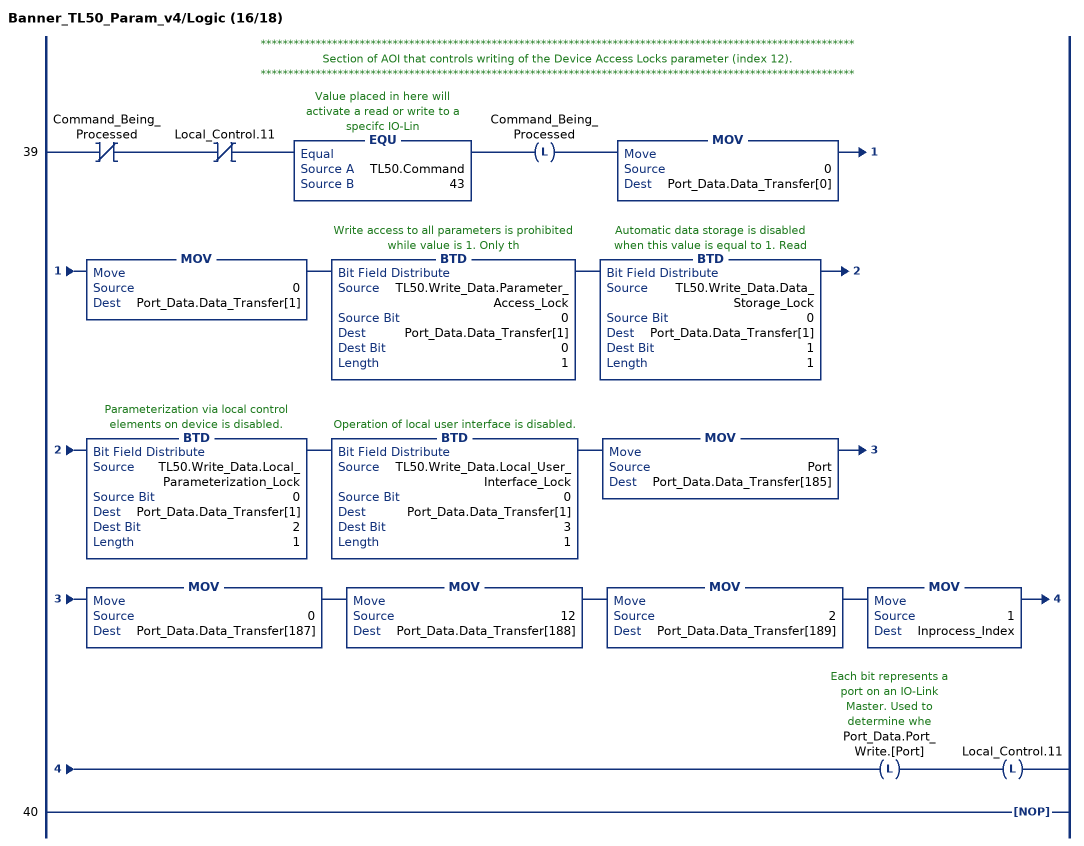
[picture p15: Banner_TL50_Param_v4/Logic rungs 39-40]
   // ************************************************************************************************************
   // Section of AOI that controls writing of the Device Access Locks parameter (index 12).
   // ************************************************************************************************************
   39: XIO(Command_Being_Processed)XIO(Local_Control.11)EQU(TL50.Command,43)OTL(Command_Being_Processed)MOV(0,Port_Data.Data_Transfer[0])MOV(0,Port_Data.Data_Transfer[1])BTD(TL50.Write_Data.Parameter_Access_Lock,0,Port_Data.Data_Transfer[1],0,1)BTD(TL50.Write_Data.Data_Storage_Lock,0,Port_Data.Data_Transfer[1],1,1)BTD(TL50.Write_Data.Local_Parameterization_Lock,0,Port_Data.Data_Transfer[1],2,1)BTD(TL50.Write_Data.Local_User_Interface_Lock,0,Port_Data.Data_Transfer[1],3,1)MOV(Port,Port_Data.Data_Transfer[185])MOV(0,Port_Data.Data_Transfer[187])MOV(12,Port_Data.Data_Transfer[188])MOV(2,Port_Data.Data_Transfer[189])MOV(1,Inprocess_Index)OTL(Port_Data.Port_Write.[Port])OTL(Local_Control.11);
   40: NOP();
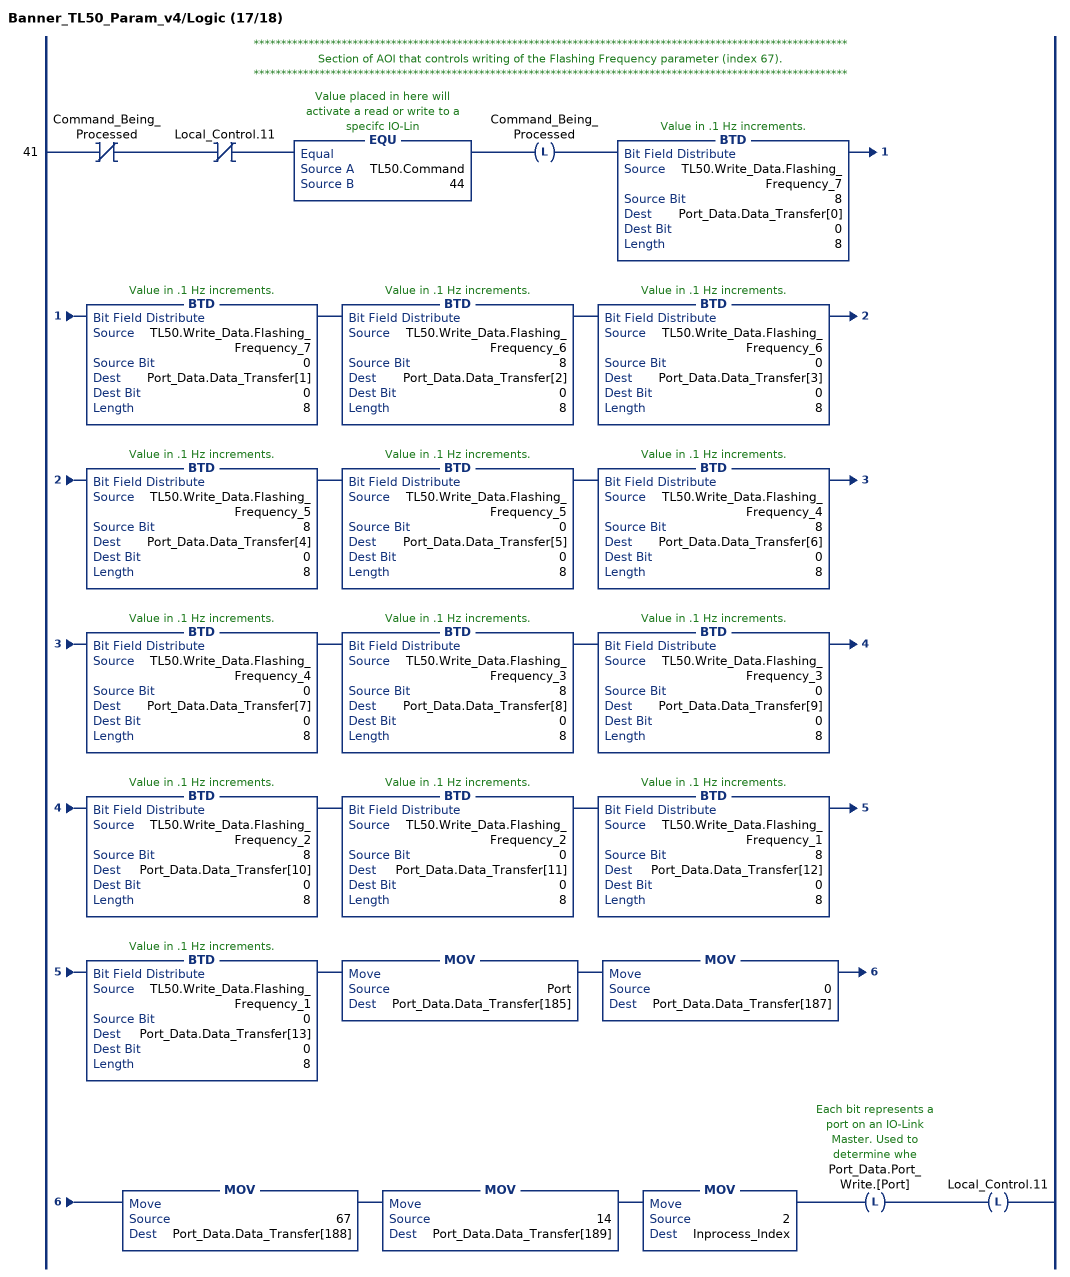
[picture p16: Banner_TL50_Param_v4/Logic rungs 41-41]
   // ************************************************************************************************************
   // Section of AOI that controls writing of the Flashing Frequency parameter (index 67).
   // ************************************************************************************************************
   41: XIO(Command_Being_Processed)XIO(Local_Control.11)EQU(TL50.Command,44)OTL(Command_Being_Processed)BTD(TL50.Write_Data.Flashing_Frequency_7,8,Port_Data.Data_Transfer[0],0,8)BTD(TL50.Write_Data.Flashing_Frequency_7,0,Port_Data.Data_Transfer[1],0,8)BTD(TL50.Write_Data.Flashing_Frequency_6,8,Port_Data.Data_Transfer[2],0,8)BTD(TL50.Write_Data.Flashing_Frequency_6,0,Port_Data.Data_Transfer[3],0,8)BTD(TL50.Write_Data.Flashing_Frequency_5,8,Port_Data.Data_Transfer[4],0,8)BTD(TL50.Write_Data.Flashing_Frequency_5,0,Port_Data.Data_Transfer[5],0,8)BTD(TL50.Write_Data.Flashing_Frequency_4,8,Port_Data.Data_Transfer[6],0,8)BTD(TL50.Write_Data.Flashing_Frequency_4,0,Port_Data.Data_Transfer[7],0,8)BTD(TL50.Write_Data.Flashing_Frequency_3,8,Port_Data.Data_Transfer[8],0,8)BTD(TL50.Write_Data.Flashing_Frequency_3,0,Port_Data.Data_Transfer[9],0,8)BTD(TL50.Write_Data.Flashing_Frequency_2,8,Port_Data.Data_Transfer[10],0,8)BTD(TL50.Write_Data.Flashing_Frequency_2,0,Port_Data.Data_Transfer[11],0,8)BTD(TL50.Write_Data.Flashing_Frequency_1,8,Port_Data.Data_Transfer[12],0,8)BTD(TL50.Write_Data.Flashing_Frequency_1,0,Port_Data.Data_Transfer[13],0,8)MOV(Port,Port_Data.Data_Transfer[185])MOV(0,Port_Data.Data_Transfer[187])MOV(67,Port_Data.Data_Transfer[188])MOV(14,Port_Data.Data_Transfer[189])MOV(2,Inprocess_Index)OTL(Port_Data.Port_Write.[Port])OTL(Local_Control.11);
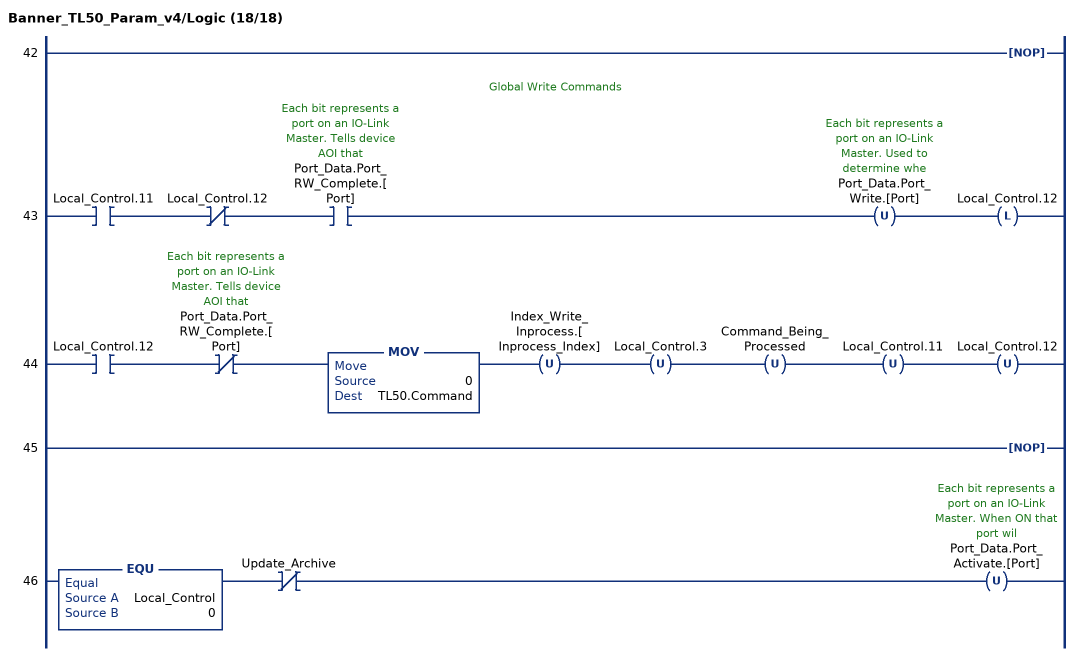
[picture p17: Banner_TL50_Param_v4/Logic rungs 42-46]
   42: NOP();
   // Global Write Commands
   43: XIC(Local_Control.11)XIO(Local_Control.12)XIC(Port_Data.Port_RW_Complete.[Port])OTU(Port_Data.Port_Write.[Port])OTL(Local_Control.12);
   44: XIC(Local_Control.12)XIO(Port_Data.Port_RW_Complete.[Port])MOV(0,TL50.Command)OTU(Index_Write_Inprocess.[Inprocess_Index])OTU(Local_Control.3)OTU(Command_Being_Processed)OTU(Local_Control.11)OTU(Local_Control.12);
   45: NOP();
   46: EQU(Local_Control,0)XIO(Update_Archive)OTU(Port_Data.Port_Activate.[Port]);
END_ROUTINE
END_ADD_ON_INSTRUCTION
